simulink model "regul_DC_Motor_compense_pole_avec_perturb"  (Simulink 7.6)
settings: Solver=ode15s  StartTime=0.0  StopTime=100  RelTol=1e-3
InitFcn:
  | clc, close all
  | k= 0.1916;
  | tau=8;
StopFcn:
  | load BO_BF_compense_pole.mat
  | plot(x(1,:),x(2,:), x(1,:),x(3,:),x(1,:),x(4,:))
  | grid
  | title('Régulation par compensation de pôle de la vitesse linéaire  du Moteur DC')
  | xlabel('temps')
  | axis([0 100 0 120])
  | 
  | figure
  | plot(x(1,:),x(5,:))
  | title('Position angulaire')
  | xlabel('temps')
  | grid
libraries: fl_lib x17, nesl_utility x6, elec_lib x1

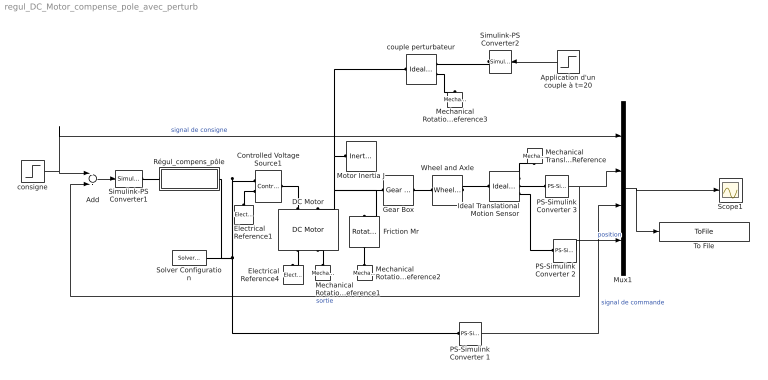
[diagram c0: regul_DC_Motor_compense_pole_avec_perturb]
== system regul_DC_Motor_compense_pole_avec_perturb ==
  Add : Sum  Inputs=+-
  Application d'un couple à t=20 : Step  Time=30  After=-2e-3  SampleTime=0
  Controlled Voltage Source1 : fl_lib/Electrical/Electrical Sources/Controlled Voltage Source  DialogController=NetworkEngine.DynNeDlgSource  SystemSampleTime=-1  i_Log=off  v_Log=off  LocalVarNames=|current|voltage|power  LocalVarDescs=|Current (A)|Voltage (V)|Power (W)  LocalVarLogging=[0 0 0]
  DC Motor : elec_lib/Actuators & Drivers/Rotational Actuators/DC Motor  DialogController=NetworkEngine.DynNeDlgSource  SystemSampleTime=-1  parameterization=1  Ra=3.9 Ohm  La=1.2e-05 H  emf_or_torque=1  Kv=7.2e-05 V/rpm  Ki=6.876e-04 N*m/A  T_stall=2.4e-04 N*m  w_max=1.91e+04 rpm  w_rated=1.5e+04 rpm  P_rated=0.08 W  V_rated=1.5 V  J=0.01 g*cm^2  lam=1e-08 N*m/(rad/s)  speed0=0 rpm  current_Log=off  voltage_Log=off  power_Log=off  i2r_Log=off  torque_Log=off  speed_Log=off  LocalVarNames=|current|voltage|power|i2r|torque|speed  LocalVarDescs=|Current (A)|Voltage (V)|Power (W)|Electrical losses (W)|Torque (Nm)|Angular speed (rad/s)  LocalVarLogging=[0 0 0 0 0 0]
  Electrical Reference1 : fl_lib/Electrical/Electrical Elements/Electrical Reference  DialogController=NetworkEngine.DynNeDlgSource  SystemSampleTime=-1  i_Log=off  LocalVarNames=|i  LocalVarDescs=|i  LocalVarLogging=[]
  Electrical Reference4 : fl_lib/Electrical/Electrical Elements/Electrical Reference  DialogController=NetworkEngine.DynNeDlgSource  SystemSampleTime=-1  i_Log=off  LocalVarNames=|i  LocalVarDescs=|i  LocalVarLogging=[]
  Friction Mr : fl_lib/Mechanical/Rotational Elements/Rotational Friction  DialogController=NetworkEngine.DynNeDlgSource  SystemSampleTime=-1  brkwy_trq=0.02e-3 N*m  Col_trq=0.02e-3 N*m  visc_coef=0 N*m/(rad/s)  trans_coef=10 s/rad  vel_thr=0.1 rad/s  t_Log=off  w_Log=off  LocalVarNames=|friction_torque|rel_velocity|power  LocalVarDescs=|Friction torque (N*m)|Relative velocity (rad/s)|Power (W)  LocalVarLogging=[0 0 0]
  Gear Box : fl_lib/Mechanical/Mechanisms/Gear Box  DialogController=NetworkEngine.DynNeDlgSource  SystemSampleTime=-1  ratio=5  t_in_Log=off  t_out_Log=off  LocalVarNames=|t_in|t_out  LocalVarDescs=|t_in|t_out  LocalVarLogging=[0 0]
  Ideal Translational Motion Sensor : fl_lib/Mechanical/Mechanical Sensors/Ideal Translational Motion Sensor  DialogController=NetworkEngine.DynNeDlgSource  SystemSampleTime=-1  offset=0 m  v_Log=off  f_Log=off  x_Log=off  LocalVarNames=|v|f|x  LocalVarDescs=|v|f|x  LocalVarLogging=[0 0 0]
  Mechanical Rotational Reference1 : fl_lib/Mechanical/Rotational Elements/Mechanical Rotational Reference  DialogController=NetworkEngine.DynNeDlgSource  SystemSampleTime=-1  t_Log=off  LocalVarNames=|t  LocalVarDescs=|t  LocalVarLogging=[]
  Mechanical Rotational Reference2 : fl_lib/Mechanical/Rotational Elements/Mechanical Rotational Reference  DialogController=NetworkEngine.DynNeDlgSource  SystemSampleTime=-1  t_Log=off  LocalVarNames=|t  LocalVarDescs=|t  LocalVarLogging=[]
  Mechanical Rotational Reference3 : fl_lib/Mechanical/Rotational Elements/Mechanical Rotational Reference  DialogController=NetworkEngine.DynNeDlgSource  SystemSampleTime=-1  t_Log=off  LocalVarNames=|t  LocalVarDescs=|t  LocalVarLogging=[]
  Mechanical Translational Reference : fl_lib/Mechanical/Translational Elements/Mechanical Translational Reference  DialogController=NetworkEngine.DynNeDlgSource  SystemSampleTime=-1  f_Log=off  LocalVarNames=|f  LocalVarDescs=|f  LocalVarLogging=0
  Motor Inertia J : fl_lib/Mechanical/Rotational Elements/Inertia  DialogController=NetworkEngine.DynNeDlgSource  SystemSampleTime=-1  inertia=10 g*cm^2  initial_velocity=0 rad/s  t_Log=off  LocalVarNames=|torque|velocity  LocalVarDescs=|Inertia torque (N*m)|Inertia absolute velocity (rad/s)  LocalVarLogging=[0 0]
  Mux1 : Mux
  PS-Simulink Converter 1 : nesl_utility/PS-Simulink Converter  DialogController=NetworkEngine.DynNeUtilDlgSource  SystemSampleTime=-1  PhysicalDomain=network_engine_domain  LeftPortType=input  RightPortType=output  SubClassName=ps_output  Unit=1  AffineConversion=off
  PS-Simulink Converter 2 : nesl_utility/PS-Simulink Converter  DialogController=NetworkEngine.DynNeUtilDlgSource  SystemSampleTime=-1  PhysicalDomain=network_engine_domain  LeftPortType=input  RightPortType=output  SubClassName=ps_output  Unit=1  AffineConversion=off
  PS-Simulink Converter 3 : nesl_utility/PS-Simulink Converter  DialogController=NetworkEngine.DynNeUtilDlgSource  SystemSampleTime=-1  PhysicalDomain=network_engine_domain  LeftPortType=input  RightPortType=output  SubClassName=ps_output  Unit=1  AffineConversion=off
  Régul_compens_pôle : Subsystem
  Scope1 : Scope
  Simulink-PS Converter1 : nesl_utility/Simulink-PS Converter  DialogController=NetworkEngine.DynNeUtilDlgSource  SystemSampleTime=-1  PhysicalDomain=network_engine_domain  LeftPortType=input  RightPortType=output  SubClassName=ps_input  Unit=1  AffineConversion=off  InputFilterTimeConstant=.001  UdotUserProvided=0
  Simulink-PS Converter2 : nesl_utility/Simulink-PS Converter  DialogController=NetworkEngine.DynNeUtilDlgSource  SystemSampleTime=-1  PhysicalDomain=network_engine_domain  LeftPortType=input  RightPortType=output  SubClassName=ps_input  Unit=1  AffineConversion=off  InputFilterTimeConstant=.001  UdotUserProvided=0
  Solver Configuration : nesl_utility/Solver Configuration  DialogController=NetworkEngine.DynNeUtilDlgSource  SystemSampleTime=-1  PhysicalDomain=network_engine_domain  LeftPortType=input  RightPortType=generic  SubClassName=solver  Accelerate=off  Profile=off  ResidualTolerance=1e-9  MaxNonlinIter=12  MaxModeIter=2  DoFixedCost=off  UseLocalSampling=off  DoDC=off  LinearAlgebra=Full  LocalSolverSampleTime=.001  LocalSolverChoice=NE_BACKWARD_EULER_ADVANCER  UseLocalSolver=off
  To File : ToFile  Filename=BO_BF_compense_pole  MatrixName=x
  Wheel and Axle : fl_lib/Mechanical/Mechanisms/Wheel and Axle  DialogController=NetworkEngine.DynNeDlgSource  SystemSampleTime=-1  R=0.05 m  or=1  torque_A_Log=off  force_P_Log=off  ang_velocity_Log=off  velocity_Log=off  LocalVarNames=|torque_A|force_P|ang_velocity|velocity  LocalVarDescs=|Axle torque (N*m)|Periphery force (N)|Axle angular velocity (rad/s)|Periphery velocity (m/s)  LocalVarLogging=[0 0 0 0]
  consigne : Step  Time=0  After=100  SampleTime=0
  couple perturbateur : fl_lib/Mechanical/Mechanical Sources/Ideal Torque Source  DialogController=NetworkEngine.DynNeDlgSource  SystemSampleTime=-1  w_Log=off  t_Log=off  LocalVarNames=|torque|rel_velocity|power  LocalVarDescs=|Torque (N*m)|Relative velocity (rad/s)|Power generated by the source (W)  LocalVarLogging=[0 0 0]
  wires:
  PS-Simulink Converter 3/1 -> Mux1/2, Add/2  "sortie"
  Add/1 -> Simulink-PS Converter1/1
  consigne/1 -> Add/1, Mux1/1  "signal de consigne"
  Mux1/1 -> To File/1, Scope1/1
  PS-Simulink Converter 1/1 -> Mux1/3  "signal de commande"
  Application d'un couple à t=20/1 -> Simulink-PS Converter2/1
  PS-Simulink Converter 2/1 -> Mux1/4  "position"
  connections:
  Ideal Translational Motion Sensor/RConn1 -- Mechanical Translational Reference/LConn1
  Mechanical Rotational Reference1/LConn1 -- DC Motor/RConn2
  Motor Inertia J/LConn1 -- Gear Box/LConn1 -- Friction Mr/LConn1 -- DC Motor/LConn2 -- couple perturbateur/LConn1
  Wheel and Axle/LConn1 -- Gear Box/RConn1
  Wheel and Axle/RConn1 -- Ideal Translational Motion Sensor/LConn1
  Friction Mr/RConn1 -- Mechanical Rotational Reference2/LConn1
  DC Motor/RConn1 -- Electrical Reference4/LConn1
  DC Motor/LConn1 -- Controlled Voltage Source1/LConn1
  Electrical Reference1/LConn1 -- Controlled Voltage Source1/RConn2
  Régul_compens_pôle/RConn1 -- Controlled Voltage Source1/RConn1 -- PS-Simulink Converter 1/LConn1 -- Solver Configuration/RConn1
  Simulink-PS Converter1/RConn1 -- Régul_compens_pôle/LConn1
  Ideal Translational Motion Sensor/RConn2 -- PS-Simulink Converter 3/LConn1
  couple perturbateur/RConn2 -- Mechanical Rotational Reference3/LConn1
  Simulink-PS Converter2/RConn1 -- couple perturbateur/RConn1
  Ideal Translational Motion Sensor/RConn3 -- PS-Simulink Converter 2/LConn1

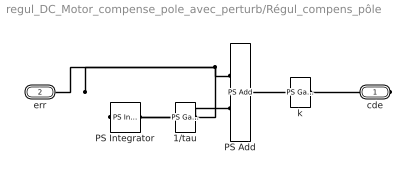
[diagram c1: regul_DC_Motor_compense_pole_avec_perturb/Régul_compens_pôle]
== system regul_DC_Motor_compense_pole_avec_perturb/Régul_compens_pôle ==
  1/tau : fl_lib/Physical Signals/Functions/PS Gain  DialogController=NetworkEngine.DynNeDlgSource  SystemSampleTime=-1  gain=1/tau  LocalVarLogging=[]
  PS Add : fl_lib/Physical Signals/Functions/PS Add  DialogController=NetworkEngine.DynNeDlgSource  SystemSampleTime=-1  LocalVarLogging=[]
  PS Integrator : fl_lib/Physical Signals/Linear Operators/PS Integrator  DialogController=NetworkEngine.DynNeDlgSource  SystemSampleTime=-1  x0=0  x_Log=off  LocalVarNames=|x  LocalVarDescs=|x  LocalVarLogging=0
  k : fl_lib/Physical Signals/Functions/PS Gain  DialogController=NetworkEngine.DynNeDlgSource  SystemSampleTime=-1  gain=k  LocalVarLogging=[]
  cde : PMIOPort  Port=1  Side=Right
  err : PMIOPort  Port=2  Side=Left
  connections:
  PS Add/RConn1 -- k/LConn1
  k/RConn1 -- cde/RConn1
  PS Integrator/RConn1 -- 1/tau/LConn1
  1/tau/RConn1 -- PS Add/LConn2
  PS Add/LConn1 -- PS Integrator/LConn1 -- err/RConn1
